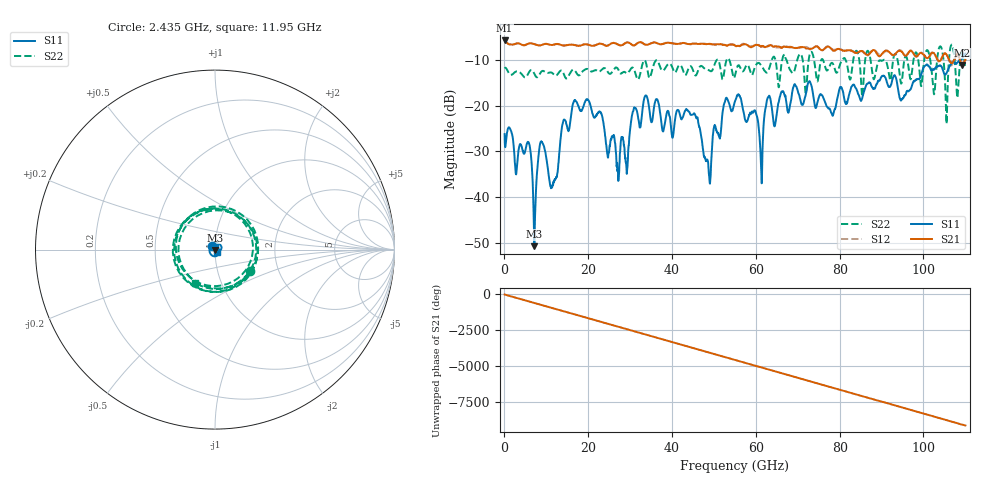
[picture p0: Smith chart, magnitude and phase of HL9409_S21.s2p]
! Created Fri Apr  1 14:40:14 2022
# ghz S ri R 50
! 2 Port Network Data from SP2.SP block
! freq  reS11  imS11  reS21  imS21  reS12  imS12  reS22  imS22
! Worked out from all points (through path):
!   2000 points, 70 MHz to 110 GHz, reference 50 ohm
!   highest |S21| = -5.75 dB at 70 MHz (marker M1); lowest = -11.1 dB at 109.2 GHz (marker M2)
!   group delay of S21, straight-line fit = 231 ps
!   lowest |S11| = -50.8 dB at 7.164 GHz (marker M3), VSWR 1.01, Z = 49.8 - j0.21 ohm
!   |S11| at or under -10 dB: start of sweep to 108.6 GHz
!   |S22| runs from -24.0 to -6.7 dB; largest |S21 - S12| = 0.028
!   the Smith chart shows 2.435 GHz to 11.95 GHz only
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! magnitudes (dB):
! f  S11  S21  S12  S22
! 70 MHz  -26.3  -5.7  -5.7  -11.6
! 5.789 GHz  -28.0  -6.4  -6.4  -12.9
! 7.164 GHz  -50.8  -6.6  -6.5  -13.0
! 8.759 GHz  -27.9  -6.8  -6.8  -12.7
! 11.45 GHz  -37.5  -6.7  -6.7  -12.9
! 14.09 GHz  -23.3  -6.9  -6.8  -12.9
! 18.44 GHz  -21.2  -6.8  -6.8  -12.8
! 27.13 GHz  -34.8  -6.7  -6.6  -12.0
! 30.98 GHz  -20.4  -6.8  -6.8  -12.1
! 36.75 GHz  -19.3  -6.4  -6.4  -10.5
! 45.66 GHz  -22.4  -6.4  -6.4  -13.4
! 48.79 GHz  -34.8  -6.5  -6.6  -12.3
! 55.06 GHz  -19.0  -6.9  -6.8  -13.3
! 61.28 GHz  -33.9  -7.1  -7.0  -11.2
! 62.98 GHz  -18.1  -7.0  -6.9  -12.4
! 73.37 GHz  -16.0  -7.5  -7.6  -8.3
! 91.69 GHz  -15.8  -8.2  -8.2  -12.7
! 102.5 GHz  -12.1  -8.6  -8.5  -17.5
! 104.1 GHz  -11.2  -10.1  -10.0  -7.0
! 105.4 GHz  -13.0  -8.7  -8.7  -22.9
! 109.2 GHz  -9.8  -11.1  -10.6  -8.4
! 110 GHz  -8.6  -10.0  -9.9  -11.8
